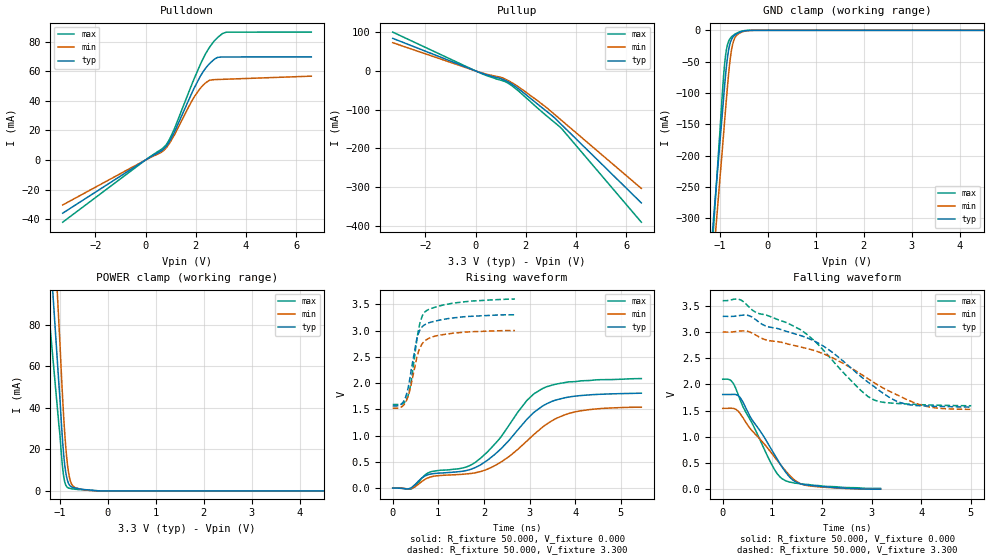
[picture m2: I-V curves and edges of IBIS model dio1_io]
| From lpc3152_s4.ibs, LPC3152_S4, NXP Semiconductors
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[Model]   dio1_io
Model_type I/O
Vinl=9.900E-01
Vinh=2.310E+00
Vref=0.000E+00
Rref=1.000E+06
Cref=2.500E-11
Vmeas=1.650E+00
C_comp   8.300E-13   8.200E-13   8.400E-13
[Voltage Range]   3.300E+00   3.000E+00   3.600E+00
[POWER Clamp Reference]   3.300E+00   3.000E+00   3.600E+00
[GND Clamp Reference]   0.000E+00   0.000E+00   0.000E+00
[Pullup Reference]   3.300E+00   3.000E+00   3.600E+00
[Pulldown Reference]   0.000E+00   0.000E+00   0.000E+00
[Temperature Range]   25   85   -40
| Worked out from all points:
|   slope of the pulldown table from 0 to 0.495 V, typ, clamps not added: 102 ohm
|   slope of the pullup table from 0 to 0.495 V, typ, clamps not added: 44.2 ohm
|   GND clamp passes 1 mA (typ) near -0.49 V on its own axis
|   POWER clamp passes 1 mA (typ) near -0.59 V on its own axis
|   rising waveform, R_fixture 50.000, V_fixture 0.000: 20-80 % time 1.38ns typ, 1.51ns min, 1.29ns max; typ from 0 V to 1.81 V
|   falling waveform, R_fixture 50.000, V_fixture 0.000: 20-80 % time 721ps typ, 810ps min, 649ps max; typ from 1.81 V to 0 V
|   rising waveform, R_fixture 50.000, V_fixture 3.300: 20-80 % time 229ps typ, 256ps min, 219ps max; typ from 1.57 V to 3.3 V
|   falling waveform, R_fixture 50.000, V_fixture 3.300: 20-80 % time 1.62ns typ, 1.86ns min, 1.44ns max; typ from 3.3 V to 1.57 V
[GND Clamp]
-3.3V     -2.286A    -2.389A    -2.834A
-1.02V    -197.6mA   -256.5mA   -185mA
-920mV    -105.7mA   -162.8mA   -70.19mA
-900mV    -87.52mA   -143.8mA   -52.73mA
-860mV    -55.24mA   -106.4mA   -29.31mA
-840mV    -42.4mA    -88.36mA   -22.49mA
-800mV    -24.47mA   -56.1mA    -14.71mA
-740mV    -12.07mA   -24.36mA   -9.185mA
-680mV    -7.188mA   -10.97mA   -5.811mA
-600mV    -3.728mA   -4.974mA   -2.713mA
-280mV    0A         0A         0A
6.6V      0A         0A         0A
[Power Clamp]
-3.3V     844.6mA    1.118A     617.8mA
-1.02V    51.26mA    80.27mA    31.64mA
-1V       44.94mA    71.65mA    27.27mA
-960mV    29.66mA    52.41mA    15.34mA
-920mV    17.25mA    35.37mA    6.877mA
-880mV    9.242mA    21.93mA    2.959mA
-860mV    6.728mA    16.66mA    2.111mA
-820mV    3.642mA    9.008mA    1.399mA
-780mV    2.297mA    4.683mA    1.162mA
-740mV    1.761mA    2.661mA    997.6uA
-380mV    435.4uA    244.8uA    267.5uA
6.6V      0A         0A         0A
[Pullup]
-3.3V     84.25mA    72.98mA    100.4mA
120mV     -2.946mA   -2.488mA   -3.578mA
1.08V     -21.97mA   -18.15mA   -25.39mA
1.24V     -26.32mA   -23.17mA   -29.71mA
1.48V     -35.59mA   -31.67mA   -39.98mA
2.82V     -103.9mA   -94.55mA   -115.8mA
3.14V     -120.9mA   -112.2mA   -133mA
3.42V     -138.8mA   -127.7mA   -148.6mA
6.6V      -341.3mA   -303.9mA   -391.2mA
[Pulldown]
-3.3V     -35.97mA   -30.41mA   -42.07mA
600mV     5.861mA    4.934mA    6.924mA
800mV     8.737mA    7.764mA    9.87mA
1.14V     18.54mA    16.66mA    20.81mA
1.86V     45.89mA    40.41mA    51.88mA
2.16V     55.95mA    48.03mA    63.81mA
2.44V     63.09mA    52.74mA    73.26mA
2.68V     67.22mA    54.27mA    79.27mA
2.86V     69.28mA    54.4mA     82.65mA
3.06V     69.64mA    54.52mA    85.46mA
3.22V     69.65mA    54.61mA    86.43mA
6.6V      69.71mA    56.67mA    86.46mA
[Rising Waveform]
R_fixture = 50.000
V_fixture = 0.000
V_fixture_min = 0.000
V_fixture_max = 0.000
|  time   V(typ)   V(min)   V(max)
0s        0V         0V         0V
410ps     9.771mV    -5.445mV   -14.73mV
790ps     259.5mV    201.1mV    295.9mV
1.54ns    322.6mV    264.5mV    384.8mV
1.79ns    385.1mV    289mV      478.9mV
2.39ns    763.7mV    505.5mV    994.5mV
2.94ns    1.309V     895.7mV    1.668V
3.33ns    1.585V     1.191V     1.914V
4.09ns    1.76V      1.468V     2.038V
5.45ns    1.808V     1.542V     2.086V
[Falling Waveform]
R_fixture = 50.000
V_fixture = 0.000
V_fixture_min = 0.000
V_fixture_max = 0.000
|  time   V(typ)   V(min)   V(max)
0s        1.808V     1.542V     2.099V
170ps     1.808V     1.545V     2.071V
260ps     1.808V     1.527V     1.932V
350ps     1.751V     1.446V     1.708V
560ps     1.372V     1.149V     1.315V
970ps     777.8mV    705.5mV    502.8mV
1.2ns     417.2mV    426.5mV    197.3mV
1.41ns    176.8mV    206.4mV    124.1mV
1.65ns    85.61mV    79mV       92.2mV
3.18ns    0V         0V         13.49mV
[Rising Waveform]
R_fixture = 50.000
V_fixture = 3.300
V_fixture_min = 3.000
V_fixture_max = 3.600
|  time   V(typ)   V(min)   V(max)
0s        1.567V     1.523V     1.593V
220ps     1.628V     1.565V     1.607V
330ps     1.877V     1.728V     1.743V
410ps     2.273V     1.996V     2.057V
530ps     2.85V      2.496V     2.831V
600ps     3.017V     2.677V     3.154V
710ps     3.115V     2.806V     3.359V
920ps     3.178V     2.893V     3.443V
1.33ns    3.242V     2.951V     3.523V
2.68ns    3.3V       3V         3.6V
[Falling Waveform]
R_fixture = 50.000
V_fixture = 3.300
V_fixture_min = 3.000
V_fixture_max = 3.600
|  time   V(typ)   V(min)   V(max)
0s        3.3V       3V         3.6V
350ps     3.317V     3.02V      3.618V
670ps     3.234V     2.941V     3.374V
1.57ns    2.933V     2.715V     3.044V
2.07ns    2.706V     2.569V     2.611V
2.75ns    2.177V     2.218V     1.915V
3.05ns    1.96V      2.035V     1.703V
3.7ns     1.621V     1.715V     1.627V
4.15ns    1.587V     1.571V     1.608V
5.01ns    1.567V     1.523V     1.593V
[Ramp]
dV/dt_r   1.0841E+00/1.3804E-09   9.2636E-01/1.5067E-09   1.2514E+00/1.2858E-09
dV/dt_f   1.0400E+00/1.6134E-09   8.8598E-01/1.8538E-09   1.2043E+00/1.4361E-09
R_load = 50
